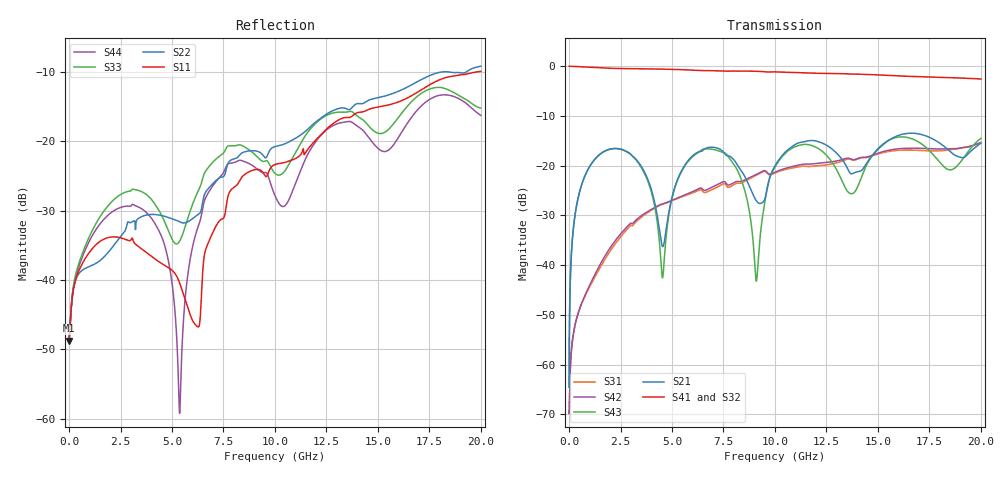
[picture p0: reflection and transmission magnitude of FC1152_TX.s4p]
! Touchstone generated by fitter/viewer
# HZ S  RI R 5.000000e+001
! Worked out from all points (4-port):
!   4999 points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, 4.001 MHz to 20 GHz, reference 50 ohm
!   strongest paths, dB at 4.001 MHz, 5.001 GHz, 10 GHz, 15 GHz, 20 GHz:
!     S41: 0.0, -0.7, -1.2, -1.8, -2.6
!     S32: 0.0, -0.7, -1.2, -1.9, -2.9
!     S21: -64.5, -26.3, -20.1, -16.7, -15.5
!     S43: -64.5, -26.6, -20.3, -16.6, -14.5
!     S42: -69.8, -27.0, -21.3, -17.5, -15.4
!     S31: -69.8, -27.0, -21.5, -17.7, -15.5
!   lowest |S11| = -48.8 dB at 4.001 MHz (marker M1), VSWR 1.01, Z = 50.4 + j0.0264 ohm
!   |S11| at or under -10 dB: start of sweep to 19.86 GHz
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4000800  0.00364 0.000262  0.000319 0.0005  -0.000314 -8.05e-05  0.9963 -0.0033
         0.000319 0.0005  0.00364 0.00028  0.9963 -0.00332  -0.000314 -8.05e-05
         -0.000314 -8.05e-05  0.9963 -0.00332  0.00364 0.000282  0.000319 0.0005
         0.9963 -0.0033  -0.000314 -8.05e-05  0.000319 0.0005  0.00364 0.000265
1.408282e9  -0.00451 -0.0179  0.1041 0.0694  -0.00693 -0.00529  0.5217 -0.8063
            0.1041 0.0694  -0.0044 -0.0127  0.5159 -0.81  -0.00716 -0.00588
            -0.00693 -0.00529  0.5159 -0.81  0.00788 -0.0259  0.1072 0.0643
            0.5217 -0.8063  -0.00716 -0.00588  0.1072 0.0643  0.00348 -0.024
4.444889e9  0.00842 0.0103  0.0164 -0.00925  -0.00395 0.0401  -0.9293 -0.062
            0.0164 -0.00925  0.0126 0.0264  -0.93 -0.0408  -0.0035 0.0404
            -0.00395 0.0401  -0.93 -0.0408  -0.0256 0.0161  0.00732 -0.00978
            -0.9293 -0.062  -0.0035 0.0404  0.00732 -0.00978  -0.0213 0.00208
5.373075e9  0.00931 0.00184  0.0511 0.0632  0.0268 0.0394  -0.7729 0.4992
            0.0511 0.0632  0.0156 0.0212  -0.7583 0.5204  0.0264 0.0405
            0.0268 0.0394  -0.7583 0.5204  0.0152 0.0116  0.0548 0.0582
            -0.7729 0.4992  0.0264 0.0405  0.0548 0.0582  0.000696 0.00085
8.881776e9  0.0603 0.0118  0.0495 -0.022  0.00974 -0.0752  0.873 0.1604
            0.0495 -0.022  0.0783 0.0338  0.8774 0.1187  0.00896 -0.077
            0.00974 -0.0752  0.8774 0.1187  -0.0836 -0.00118  -0.00633 -0.0217
            0.873 0.1604  0.00896 -0.077  -0.00633 -0.0217  -0.0645 -0.0185
1.356671e10  0.1378 -0.0537  0.078 -0.0439  0.0138 0.1159  -0.8244 -0.1062
             0.078 -0.0439  0.1648 -0.0365  -0.8181 -0.0372  0.0169 0.1173
             0.0138 0.1159  -0.8181 -0.0372  -0.1539 -0.0539  -0.0485 -0.0232
             -0.8244 -0.1062  0.0169 0.1173  -0.0485 -0.0232  -0.118 -0.0726
2e10  0.1481 -0.2819  0.129 -0.1074  -0.1679 -0.00543  0.3284 -0.6637
      0.129 -0.1074  0.1634 -0.3059  0.2341 -0.6811  -0.1705 -0.00703
      -0.1679 -0.00543  0.2341 -0.6811  0.024 0.1714  0.1482 0.1154
      0.3284 -0.6637  -0.1705 -0.00703  0.1482 0.1154  -0.0309 0.1502
